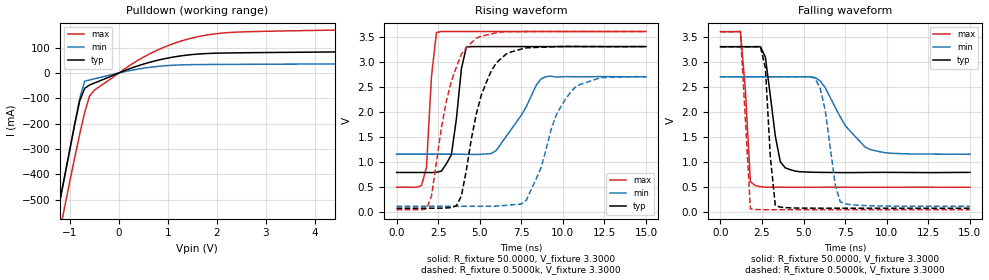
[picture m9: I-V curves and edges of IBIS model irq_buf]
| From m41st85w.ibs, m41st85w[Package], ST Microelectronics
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|   Model irq_buf
[Model]   irq_buf
Model_type   Open_drain
Polarity   Inverting
Vmeas =   1.5000V
Cref =  50.0000pF
Rref =   0.3330k
Vref =   1.7300V
C_comp   4.5500pF   4.4200pF   4.6300pF
[Temperature Range]   27.0000   85.0000   -40.0000
[Voltage Range]   3.2000V   2.7000V   3.6000V
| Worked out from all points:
|   slope of the pulldown table from 0 to 0.48 V, typ, clamps not added: 14.3 ohm
|   rising waveform, R_fixture 50.0000, V_fixture 3.3000: 20-80 % time 521ps typ, 1.7ns min, 357ps max; typ from 0.793 V to 3.3 V
|   rising waveform, R_fixture 0.5000k, V_fixture 3.3000: 20-80 % time 1.36ns typ, 1.68ns min, 1.3ns max; typ from 0.081 V to 3.3 V
|   falling waveform, R_fixture 50.0000, V_fixture 3.3000: 20-80 % time 615ps typ, 1.78ns min, 356ps max; typ from 3.3 V to 0.795 V
|   falling waveform, R_fixture 0.5000k, V_fixture 3.3000: 20-80 % time 379ps typ, 669ps min, 361ps max; typ from 3.3 V to 0.081 V
[Pulldown]
| voltage   I(typ)   I(min)   I(max)
-3.2V     -2.5A      -2.5A      -2.586A
-1.4V     -700mA     -700mA     -810.5mA
-1V       -300mA     -300mA     -425.7mA
-800mV    -109.6mA   -100mA     -241.4mA
-700mV    -61.27mA   -32.57mA   -156.4mA
-600mV    -47.64mA   -27.79mA   -91.21mA
-500mV    -39.89mA   -23.29mA   -67.59mA
100mV     7.894mA    4.371mA    13.86mA
800mV     50.46mA    25.78mA    91.43mA
1.5V      72.58mA    32.65mA    138.2mA
2.5V      79.48mA    33.9mA     161.8mA
6.4V      86.87mA    37.52mA    176.6mA
[Ramp]
| variable   typ   min   max
dV/dt_r   1.8493/0.9042n   1.5128/1.0653n   2.1145/0.8614n
dV/dt_f   1.8493/0.2965n   1.5128/0.6915n   2.1149/0.1935n
R_load = 0.3330k
[Rising Waveform]
R_fixture = 50.0000
V_fixture = 3.3000
V_fixture_min = 2.7000
V_fixture_max = 3.6000
| time   V(typ)   V(min)   V(max)
0s        793mV      1.158V     498.3mV
1.5ns     793mV      1.158V     530.9mV
1.8ns     792.3mV    1.158V     892.5mV
2.1ns     790.6mV    1.158V     2.704V
2.4ns     796.9mV    1.158V     3.58V
3.3ns     1.149V     1.159V     3.6V
4.2ns     3.292V     1.154V     3.6V
6ns       3.3V       1.234V     3.6V
9ns       3.3V       2.702V     3.6V
15ns      3.3V       2.698V     3.6V
[Rising Waveform]
R_fixture = 0.5000k
V_fixture = 3.3000
V_fixture_min = 2.7000
V_fixture_max = 3.6000
| time   V(typ)   V(min)   V(max)
0s        81.1mV     119mV      50.58mV
1.8ns     81.14mV    119mV      69.9mV
3.6ns     130.8mV    119mV      2.892V
4.8ns     1.963V     118.6mV    3.47V
5.7ns     2.818V     119.2mV    3.552V
6.9ns     3.193V     147.3mV    3.597V
7.8ns     3.274V     239.8mV    3.599V
9.6ns     3.299V     1.934V     3.6V
10.8ns    3.303V     2.506V     3.6V
15ns      3.3V       2.7V       3.6V
[Falling Waveform]
R_fixture = 50.0000
V_fixture = 3.3000
V_fixture_min = 2.7000
V_fixture_max = 3.6000
| time   V(typ)   V(min)   V(max)
0s        3.3V       2.7V       3.6V
1.2ns     3.3V       2.7V       3.602V
1.8ns     3.3V       2.7V       610.1mV
2.1ns     3.3V       2.7V       531mV
2.7ns     3.093V     2.7V       499.6mV
3.3ns     1.515V     2.7V       498.6mV
3.9ns     884.5mV    2.7V       498.4mV
6ns       795.1mV    2.619V     498.4mV
9ns       793.8mV    1.251V     497.9mV
15ns      795.4mV    1.159V     497.9mV
[Falling Waveform]
R_fixture = 0.5000k
V_fixture = 3.3000
V_fixture_min = 2.7000
V_fixture_max = 3.6000
| time   V(typ)   V(min)   V(max)
0s        3.3V       2.7V       3.6V
1.2ns     3.3V       2.7V       3.603V
1.8ns     3.3V       2.7V       67.08mV
2.7ns     2.882V     2.7V       51.03mV
3ns       1.103V     2.7V       49.93mV
3.3ns     132.1mV    2.7V       50.27mV
5.7ns     81.16mV    2.664V     50.01mV
6.3ns     81.15mV    2.034V     50.42mV
7.2ns     81.14mV    211.6mV    51.04mV
15ns      81.04mV    118.9mV    49.98mV
